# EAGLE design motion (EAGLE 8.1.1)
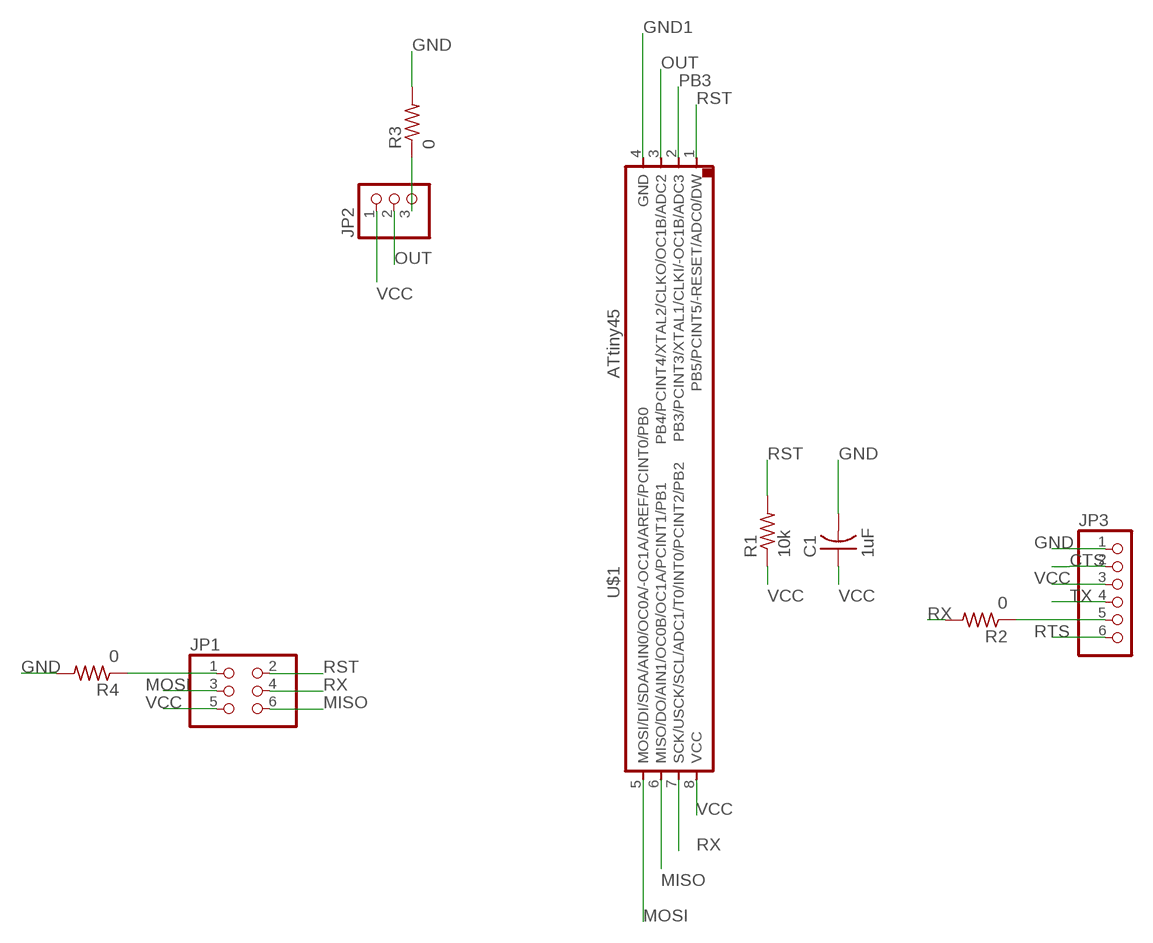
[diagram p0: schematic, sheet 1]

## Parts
C1  1uF  CAP-US1206FAB  [C1206FAB]
JP1  PINHD-2X3-SMD  [2X03SMD]
JP2  PINHD-1X3  [1X03]
JP3  PINHD-1X6  [1X06]
R1  10k  RES-US1206FAB  [R1206FAB]
R2  0  RES-US1206FAB  [R1206FAB]
R3  0  RES-US1206FAB  [R1206FAB]
R4  0  RES-US1206FAB  [R1206FAB]
U$1  ATTINY45SI  [SOIC8]

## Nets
CTS: JP3.2
GND: C1.2 JP3.1 R3.2 R4.2
GND1: JP1.1 R4.1 U$1.4(GND)
MISO: JP1.6 U$1.6(MISO/DO/AIN1/OC0B/OC1A/PCINT1/PB1)
MOSI: JP1.3 U$1.5(MOSI/DI/SDA/AIN0/OC0A/-OC1A/AREF/PCINT0/PB0)
N$1: JP3.5 R2.1
N$2: JP2.3 R3.1
OUT: JP2.2 U$1.3(PB4/PCINT4/XTAL2/CLKO/OC1B/ADC2)
PB3: U$1.2(PB3/PCINT3/XTAL1/CLKI/-OC1B/ADC3)
RST: JP1.2 R1.2 U$1.1(PB5/PCINT5/-RESET/ADC0/DW)
RTS: JP3.6
RX: JP1.4 R2.2 U$1.7(SCK/USCK/SCL/ADC1/T0/INT0/PCINT2/PB2)
TX: JP3.4
VCC: C1.1 JP1.5 JP2.1 JP3.3 R1.1 U$1.8(VCC)

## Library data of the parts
C1 = fab:CAP-US
JP1 = fab:PINHD-2X3-SMD: PIN HEADER
JP2 = pinhead:PINHD-1X3: PIN HEADER
JP3 = pinhead:PINHD-1X6: PIN HEADER
R1-R4 = fab:RES-US: Resistor (US Symbol)
U$1 = fab:ATTINY45

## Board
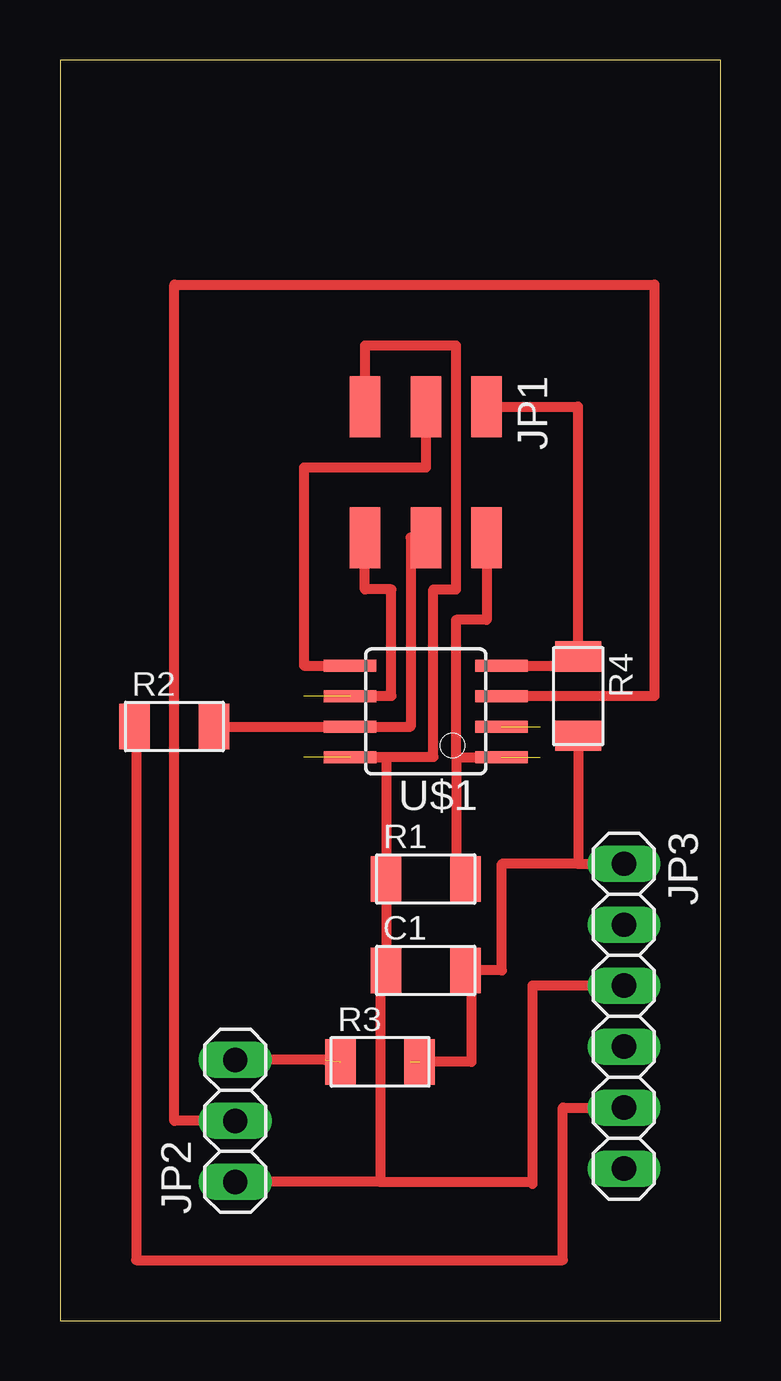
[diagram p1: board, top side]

Size 27.54 x 52.54 mm. Coordinates in mm from the lower left corner, seen from the top.
Outline: 0,0 27.54,0 27.54,52.54 0,52.54 0,0
Copper layers (1*16): Top 0.035mm / dielectric 1.5mm / Bottom 0.035mm
Design rules "default *": minimum track width 10mil, minimum drill 24mil, track to track 0.4mm, track to pad 0.4mm, pad to pad 0.4mm, via to via 0.4mm, smd to smd 0.4mm, copper to edge 40mil, drill to drill 8mil, minimum pad ring 10mil, minimum via ring 8mil, stop-mask expansion 4mil, vias tented up to drill 0mil, thermal gap 10mil

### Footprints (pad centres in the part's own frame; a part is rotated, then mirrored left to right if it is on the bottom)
C1206FAB = smd 1.27 x 1.905: 1 -1.651,0; 2 1.651,0
2X03SMD = smd 2.54 x 1.27: 1 -2.54,2.54; 2 2.92,2.54; 3 -2.54,0; 4 2.92,0; 5 -2.54,-2.54; 6 2.92,-2.54
1X03 = drill 1.016 long: 1 -2.54,0; 2 0,0; 3 2.54,0
1X06 = drill 1.016 long: 1 -6.35,0; 2 -3.81,0; 3 -1.27,0; 4 1.27,0; 5 3.81,0; 6 6.35,0
R1206FAB = smd 1.27 x 1.905: 1 -1.651,0; 2 1.651,0
SOIC8 = smd 0.5 x 2.2: 1 -1.905,-3.154; 2 -0.645,-3.154; 3 0.625,-3.154; 4 1.895,-3.154; 5 1.905,3.154; 6 0.635,3.154; 7 -0.635,3.154; 8 -1.905,3.154

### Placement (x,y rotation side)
C1  15.24,14.61 0 top
JP1  15.24,35.56 270 top
JP2  7.3,8.34 90 top
JP3  23.5,12.7 270 top
R1  15.24,18.41 0 top
R2  4.76,24.77 0 top
R3  13.34,10.79 0 top
R4  21.59,26.04 270 top
U$1  15.24,25.4 90 top

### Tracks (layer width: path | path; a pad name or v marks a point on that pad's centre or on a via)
GND  (1 unrouted)
  Top 0.406: 21.59,19.05 18.41,19.05 18.41,14.61 C1.2 17.14,14.61 17.14,10.79 14.61,10.79 | 21.59,19.05 JP3.1 | R4.2 21.59,19.05
GND1
  Top 0.406: JP1.1 21.59,38.1 R4.1 21.59,27.3 U$1.4
MISO  (1 unrouted)
  Top 0.406: U$1.6 13.81,26.04 13.81,30.48 12.7,30.48 JP1.6
MOSI
  Top 0.406: JP1.3 15.24,35.56 10.16,35.56 10.16,27.3 U$1.5
N$1
  Top 0.406: R2.1 3.17,24.77 3.17,2.54 20.95,2.54 20.95,8.89 JP3.5
N$2  (1 unrouted)
  Top 0.406: 11.05,10.88 JP2.3
OUT
  Top 0.406: JP2.2 4.76,8.34 4.76,43.18 24.77,43.18 24.77,26.04 18.39,26.04 U$1.3
PB3  (2 unrouted)
RST  (1 unrouted)
  Top 0.406: JP1.2 17.78,29.21 16.51,29.21 16.51,23.5 | 16.51,23.5 16.51,19.05 16.89,19.05 R1.2 | 16.51,23.5 U$1.1
RX
  Top 0.406: JP1.4 14.61,32.64 14.61,24.77 U$1.7 R2.2
VCC  (1 unrouted)
  Top 0.406: JP1.5 12.7,40.64 16.51,40.64 16.51,30.48 15.56,30.48 15.56,23.5 U$1.8 13.59,23.5 R1.1 C1.1 13.34,14.61 13.34,5.79 | 13.34,5.79 19.68,5.79 | 13.34,5.79 JP2.1 | 19.68,5.79 19.68,5.71 | JP3.3 19.68,13.97 19.68,5.79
